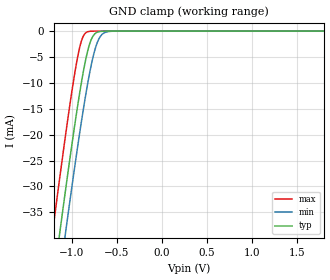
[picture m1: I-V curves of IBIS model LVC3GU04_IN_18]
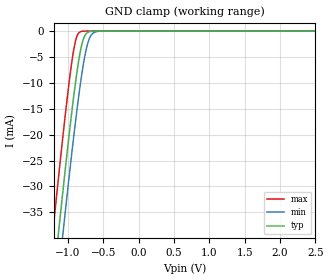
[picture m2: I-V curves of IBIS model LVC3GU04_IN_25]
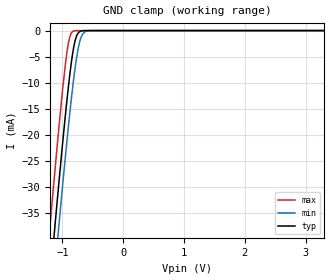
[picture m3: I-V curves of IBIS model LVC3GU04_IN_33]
| TEXAS INSTRUMENTS INCORPORATED
| Standard Linear and Logic Group
| IBIS Model of SN74LVC3GU04
| TRIPLE INVERTER GATE
| This file contains package information for the following:
|  SSOP 8-pin (DCT) package as [Component] LVC3GU04_DCT
|  VSSOP 8-pin (DCU) package as [Component] LVC3GU04_DCU
|  NanoStar WCSP 8-pin (YEA) package as [Component] LVC3GU04_YEP
|  NanoFree WCSP 8-pin (YZA) package as [Component] LVC3GU04_YZP
| This device can be powered at the following Vccs:
|  1.8 volt Vcc
|  2.5 volt Vcc
|  3.3 volt Vcc
|  5 volt Vcc
| This file provides unique models under the [Model Selector] for each Vcc.
| For operation at a specific Vcc, select the appropriate model after each
| [Model Selector] keyword.
[IBIS Ver]   3.2
[Comment char]  |_char
[File Name]   sn74lvc3gu04.ibs
[File Rev]   1.3 | e_die
[Date]   February 10, 2004
[Source]   Data created from TI-SPICE simulations at TI-SLL.
[Notes]   The following is an IBIS list for the SN74LVC3GU04.
   Please contact sllibis@ti.com with questions and
   comments concerning SLL IBIS models.
   - FILE REV HISTORY
   - 1.2 added YEP and YZP packages on 02/04/04
   - 1.3 Die rev correction on 02/10/04
   - C_comp values are taken at a different test condition than
   the Ci in data sheet.
   - Power-clamp data has been deleted since there is no
   power-clamp diode in the device.
[Disclaimer] Property of Texas Instruments Incorporated. Unauthorized
   reproduction and/or distribution is strictly prohibited.
   This product is protected under copyright law.
   Created 2003,(C) Copyright 2003, Texas Instruments
   Incorporated, All Rights Reserved
   UNLESS THERE IS A SIGNED, WRITTEN AGREEMENT TO THE
   CONTRARY, TEXAS INSTRUMENTS (TI) IS PROVIDING THE IBIS
   MODELS AND WITHOUT ANY WARRANTY, EXPRESSED OR
   IMPLIED. TI assumes no liability for:
   1) the accuracy of the IBIS models provided to your
   company;
   2) the proper functioning of these IBIS Models in your
   design or for any resulting applications; or
   3) infringement of patents, copyrights or intellectual
   property rights resulting from your use of these IBIS
   models.
   TI provides IBIS Models as a service to our customers.
   You and your company shall not distribute, sell or give
   these models to anyone else without prior written
   permission from TI.
   TI reserves the right to make changes to our products or
   to discontinue any semiconductor product or service
   without notice, and advises our customers to obtain the
   latest version of relevant information to verify, before
   placing orders, that the information being relied on is
   current.
   Please be aware that your receipt and use of the IBIS
   information provided shall serve as acceptance of these
   terms and conditions. If you do not accept these terms,
   you should return or destroy the IBIS models and any
   other accompanying information immediately.
| Component LVC3GU04_DCT 8-pin SSOP
[Component]   LVC3GU04_DCT
[Manufacturer]   Texas Instruments, Inc.
[Package]
|   typ   min   max
R_pkg   2.900e-02   2.800e-02   3.100e-02
L_pkg   1.796e-09   1.666e-09   1.924e-09
C_pkg   1.090e-13   8.300e-14   1.360e-13
[Pin]   signal_name   model_name   R_pin   L_pin   C_pin
1   1A   LVC3GU04_IN   3.100e-02   1.894e-09   1.340e-13
2   3Y   LVC3GU04_OUT   2.800e-02   1.697e-09   8.600e-14
3   2A   LVC3GU04_IN   3.000e-02   1.722e-09   8.600e-14
4   GND   GND   3.000e-02   1.861e-09   1.300e-13
5   2Y   LVC3GU04_OUT   2.800e-02   1.924e-09   1.360e-13
6   3A   LVC3GU04_IN   2.900e-02   1.736e-09   8.600e-14
7   1Y   LVC3GU04_OUT   2.800e-02   1.666e-09   8.300e-14
8   VCC   POWER   3.000e-02   1.871e-09   1.320e-13
| Component LVC3GU04_DCU 8-pin VSSOP
[Component]   LVC3GU04_DCU
[Manufacturer]   Texas Instruments, Inc.
[Package]
|   typ   min   max
R_pkg   2.600e-02   2.300e-02   3.800e-02
L_pkg   1.394e-09   1.066e-09   2.046e-09
C_pkg   2.590e-13   2.150e-13   3.720e-13
[Pin]   signal_name   model_name   R_pin   L_pin   C_pin
1   1A   LVC3GU04_IN   2.400e-02   1.520e-09   2.710e-13
2   3Y   LVC3GU04_OUT   2.300e-02   1.112e-09   2.180e-13
3   2A   LVC3GU04_IN   2.300e-02   1.070e-09   2.170e-13
4   GND   GND   2.700e-02   2.046e-09   3.720e-13
5   2Y   LVC3GU04_OUT   2.700e-02   1.542e-09   2.730e-13
6   3A   LVC3GU04_IN   2.300e-02   1.100e-09   2.240e-13
7   1Y   LVC3GU04_OUT   2.300e-02   1.066e-09   2.150e-13
8   VCC   POWER   3.800e-02   1.696e-09   2.800e-13
| Component LVC3GU04_YEP 8-pin DSBGA
[Component]   LVC3GU04_YEP
[Manufacturer]   Texas Instruments, Inc.
[Package]
|   typ   min   max
R_pkg   1.000e-03   1.000e-03   1.000e-03
L_pkg   2.450e-11   2.400e-11   2.500e-11
C_pkg   6.550e-14   6.400e-14   6.700e-14
[Pin]   signal_name   model_name   R_pin   L_pin   C_pin
1   1A   LVC3GU04_IN   1.000e-03   2.500e-11   6.400e-14
2   3Y   LVC3GU04_OUT   1.000e-03   2.400e-11   6.700e-14
3   2A   LVC3GU04_IN   1.000e-03   2.400e-11   6.700e-14
4   GND   GND   1.000e-03   2.500e-11   6.400e-14
5   2Y   LVC3GU04_OUT   1.000e-03   2.500e-11   6.400e-14
6   3A   LVC3GU04_IN   1.000e-03   2.400e-11   6.700e-14
7   1Y   LVC3GU04_OUT   1.000e-03   2.400e-11   6.700e-14
8   VCC   POWER   1.000e-03   2.500e-11   6.400e-14
| Component LVC3GU04_YZP 8-pin DSBGA
[Component]   LVC3GU04_YZP
[Manufacturer]   Texas Instruments, Inc.
[Package]
|   typ   min   max
R_pkg   1.000e-03   1.000e-03   1.000e-03
L_pkg   2.450e-11   2.400e-11   2.500e-11
C_pkg   6.550e-14   6.400e-14   6.700e-14
[Pin]   signal_name   model_name   R_pin   L_pin   C_pin
1   1A   LVC3GU04_IN   1.000e-03   2.500e-11   6.400e-14
2   3Y   LVC3GU04_OUT   1.000e-03   2.400e-11   6.700e-14
3   2A   LVC3GU04_IN   1.000e-03   2.400e-11   6.700e-14
4   GND   GND   1.000e-03   2.500e-11   6.400e-14
5   2Y   LVC3GU04_OUT   1.000e-03   2.500e-11   6.400e-14
6   3A   LVC3GU04_IN   1.000e-03   2.400e-11   6.700e-14
7   1Y   LVC3GU04_OUT   1.000e-03   2.400e-11   6.700e-14
8   VCC   POWER   1.000e-03   2.500e-11   6.400e-14
| Model LVC3GU04_IN
[Model Selector]   LVC3GU04_IN
LVC3GU04_IN_18   1.8 volt Vcc
LVC3GU04_IN_25   2.5 volt Vcc
LVC3GU04_IN_33   3.3 volt Vcc
LVC3GU04_IN_50   5 volt Vcc
| Model LVC3GU04_OUT
[Model Selector]   LVC3GU04_OUT
LVC3GU04_OUT_18   1.8 volt Vcc
LVC3GU04_OUT_25   2.5 volt Vcc
LVC3GU04_OUT_33   3.3 volt Vcc
LVC3GU04_OUT_50   5 volt Vcc
| Models and submodels in the file (8): LVC3GU04_IN_18 (Input), LVC3GU04_IN_25 (Input), LVC3GU04_IN_33 (Input), LVC3GU04_IN_50 (Input), LVC3GU04_OUT_18 (Output), LVC3GU04_OUT_25 (Output), LVC3GU04_OUT_33 (Output), LVC3GU04_OUT_50 (Output)
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[Model]   LVC3GU04_IN_18
Model_type  Input
Vinl=0.4125
Vinh=1.4625
| variable   typ   min   max
C_comp   5.94pF   3.50pF   6.92pF
[Temperature Range]   40   100   -40
| Ambient temperature   25   85   -40
[Voltage range]   1.8   1.65   1.95
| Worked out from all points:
|   GND clamp passes 1 mA (typ) near -0.77 V on its own axis
[GND Clamp]
| LVC3GU04_IN_18
|   Voltage   I(typ)   I(min)   I(max)
-5.5V     -655.2mA   -662.2mA   -646.6mA
-1.215V   -49.6mA    -57.88mA   -38.96mA
-1.135V   -39.07mA   -47.36mA   -28.42mA
-1.075V   -31.35mA   -39.6mA    -20.75mA
-1.055V   -28.82mA   -37.05mA   -18.27mA
-955mV    -16.68mA   -24.66mA   -6.874mA
-885mV    -9.098mA   -16.55mA   -1.486mA
-825mV    -3.922mA   -10.26mA   -137.1uA
-780mV    -1.472mA   -6.227mA   -17.15uA
-715mV    -205.4uA   -2.128mA   -808.5nA
-650mV    -22.01uA   -443.9uA   -37.93nA
1.8V      3.326pA    6.142pA    3.026pA
[Model]   LVC3GU04_IN_25
Model_type  Input
Vinl=0.575
Vinh=2.025
| variable   typ   min   max
C_comp   6.25pF   4.07pF   7.77pF
[Temperature Range]   40   100   -40
| Ambient temperature   25   85   -40
[Voltage range]   2.5   2.3   2.7
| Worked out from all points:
|   GND clamp passes 1 mA (typ) near -0.77 V on its own axis
[GND Clamp]
| LVC3GU04_IN_25
|   Voltage   I(typ)   I(min)   I(max)
-5.5V     -655.2mA   -662.2mA   -646.6mA
-1.215V   -49.6mA    -57.88mA   -38.96mA
-1.14V    -39.72mA   -48.01mA   -29.07mA
-1.12V    -37.12mA   -45.41mA   -26.48mA
-1.08V    -31.98mA   -40.25mA   -21.38mA
-1.06V    -29.44mA   -37.69mA   -18.89mA
-960mV    -17.26mA   -25.26mA   -7.377mA
-890mV    -9.597mA   -17.1mA    -1.734mA
-785mV    -1.671mA   -6.635mA   -21.67uA
-720mV    -242.5uA   -2.354mA   -1.023uA
-650mV    -22.01uA   -443.9uA   -37.93nA
2.5V      4.713pA    7.577pA    4.389pA
[Model]   LVC3GU04_IN_33
Model_type  Input
Vinl=0.75
Vinh=2.7
| variable   typ   min   max
C_comp   6.37pF   4.31pF   7.88pF
[Temperature Range]   40   100   -40
| Ambient temperature   25   85   -40
[Voltage range]   3.3   3   3.6
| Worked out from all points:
|   GND clamp passes 1 mA (typ) near -0.77 V on its own axis
[GND Clamp]
| LVC3GU04_IN_33
|   Voltage   I(typ)   I(min)   I(max)
-5.5V     -655.2mA   -662.2mA   -646.6mA
-1.225V   -50.93mA   -59.21mA   -40.3mA
-1.145V   -40.37mA   -48.66mA   -29.72mA
-1.12V    -37.12mA   -45.41mA   -26.48mA
-1.08V    -31.98mA   -40.25mA   -21.38mA
-1.06V    -29.44mA   -37.69mA   -18.89mA
-965mV    -17.84mA   -25.87mA   -7.89mA
-885mV    -9.098mA   -16.55mA   -1.486mA
-780mV    -1.472mA   -6.227mA   -17.15uA
-715mV    -205.4uA   -2.128mA   -808.5nA
-640mV    -15.53uA   -338.1uA   -23.69nA
3.3V      6.304pA    9.258pA    5.93pA
